|   TEXAS INSTRUMENTS INCORPORATED
|   Standard Linear and Logic
|   IBIS Model of SN74LVTH162241
|   3.3-V ABT 16-BIT BUFFERS/DRIVERS
|   WITH 3-STATE OUTPUTS
|   TSSOP 48-pin package (DGG)
|   SSOP 48-pin package (DL)
[IBIS Ver]   3.2
[Comment char] |_char
[File Name]   sn74lvth162241.ibs
[File Rev]   1.1 | a_die
[Date]   04/12/02
[Source]   File originated at Texas Instruments, Inc
[Notes]   The following is a sample IBIS file for the SNLVTH162241.
   - All test data contained in this file are derived from
   actual measurement.
   - The measurement used DGG package.
   - We have data across voltage and temperature, but not across
   process.
   - Since this is a BiCMOS process, we have irregular trend for the
   curves at high and low temperatures. This data was taken with
   high temperature for strong case and low for weak case.
   - Due to presence of BUS-HOLD at input, GND-CLAMP curves
   have non-monotonic warnings.
   - File created by Nobuhisa Ohtsubo, TIJ SLL Product Engineering.
   - We ommitted some Pwr_Clamp data as there is no Power
   clamp diode at the input
   - Due to 5V tollerant circuitry, we have non-monotonic warnings
   at the pull-up curves
|*   Property of Texas Instruments Incorporated.  Unauthorized   *
|*   reproduction and/or distribution is strictly prohibited.   *
|*   This product is protected under copyright law.   *
|*   Created 1998, (C) Copyright 1998, Texas Instruments Inc.,   *
|*   All Rights Reserved   *
|*   UNLESS THERE IS A SIGNED, WRITTEN AGREEMENT TO THE   *
|*   CONTRARY, TEXAS INSTRUMENTS ("TI") IS PROVIDING THE SPICE   *
|*   MODELS "AS IS" AND WITHOUT ANY WARRANTY, EXPRESSED OR   *
|*   IMPLIED.  TI assumes no liability for:   *
|*   1) the accuracy of the IBIS models provided to your   *
|*   company;   *
|*   2) the proper functioning of these IBIS models in your   *
|*   design or for any resulting applications; or   *
|*   3) infringement of patents, copyrights or intellectual   *
|*   property rights resulting from your use of these   *
|*   IBIS models.   *
|*   TI provides IBIS Models as a service to our customers.   *
|*   You and your company shall not distribute, sell or give   *
|*   these models to anyone else without prior written   *
|*   permission from TI.   *
|*   TI reserves the right to make changes to our products or   *
|*   to discontinue any semiconductor product or service   *
|*   without notice, and advises our customers to obtain the   *
|*   latest version of relevant information to verify, before   *
|*   placing orders, that the information being relied on is   *
|*   current.   *
|*   Please be aware that your receipt and use of the IBIS   *
|*   information provided shall serve as acceptance of these   *
|*   terms and conditions.  If you do not accept these terms,   *
|*   you should return or destroy the IBIS models and any   *
|*   other accompanying information immediately.   *
|   TSSOP PACKAGE (DGG)
[Component]   LVTH162241_DGG
[manufacturer]   Texas Instruments, Inc.
[Package]
|   typ   min   max
R_pkg   0.044   0.038   0.051
L_pkg   3.019nH   2.486nH   4.099nH
C_pkg   0.507pF   0.334pF   0.809pF
[Pin] signal_name   model_name   R_pin   L_pin   C_pin
1   1NOE   LVTH162241_OE   0.041   4.017nH   0.759pF
2   1Y1   LVTH162241_OUT  0.042   3.737nH   0.792pF
3   1Y2   LVTH162241_OUT  0.042   3.48nH   0.661pF
4   GND   GND   0.038   3.131nH   0.575pF
5   1Y3   LVTH162241_OUT  0.047   3.122nH   0.566pF
6   1Y4   LVTH162241_OUT  0.043   2.948nH   0.504pF
7   VCC   POWER   0.045   2.845nH   0.397pF
8   2Y1   LVTH162241_OUT  0.049   2.835nH   0.394pF
9   2Y2   LVTH162241_OUT  0.048   2.715nH   0.378pF
10   GND   GND   0.050   2.664nH   0.363pF
11   2Y3   LVTH162241_OUT  0.050   2.585nH   0.348pF
12   2Y4   LVTH162241_OUT  0.049   2.55nH   0.337pF
13   3Y1   LVTH162241_OUT  0.049   2.541nH   0.336pF
14   3Y2   LVTH162241_OUT  0.050   2.574nH   0.348pF
15   GND   GND   0.049   2.618nH   0.359pF
16   3Y3   LVTH162241_OUT  0.046   2.671nH   0.375pF
17   3Y4   LVTH162241_OUT  0.045   2.754nH   0.389pF
18   VCC   POWER   0.044   2.823nH   0.450pF
19   4Y1   LVTH162241_OUT  0.042   2.968nH   0.503pF
20   4Y2   LVTH162241_OUT  0.051   3.108nH   0.535pF
21   GND   GND   0.042   3.175nH   0.587pF
22   4Y3   LVTH162241_OUT  0.041   3.449nH   0.678pF
23   4Y4   LVTH162241_OUT  0.044   3.766nH   0.804pF
24   4NOE   LVTH162241_OE   0.043   4.065nH   0.761pF
25   3OE   LVTH162241_OE   0.041   3.994nH   0.757pF
26   4A4   LVTH162241_IN   0.039   3.649nH   0.789pF
27   4A3   LVTH162241_IN   0.038   3.362nH   0.660pF
28   GND   GND   0.038   3.082nH   0.574pF
29   4A2   LVTH162241_IN   0.044   2.99nH   0.522pF
30   4A1   LVTH162241_IN   0.041   2.917nH   0.495pF
31   VCC   POWER   0.043   2.82nH   0.448pF
32   3A4   LVTH162241_IN   0.043   2.699nH   0.385pF
33   3A3   LVTH162241_IN   0.045   2.628nH   0.372pF
34   GND   GND   0.046   2.556nH   0.356pF
35   3A2   LVTH162241_IN   0.046   2.495nH   0.344pF
36   3A1   LVTH162241_IN   0.047   2.487nH   0.334pF
37   2A4   LVTH162241_IN   0.047   2.49nH   0.335pF
38   2A3   LVTH162241_IN   0.046   2.486nH   0.343pF
39   GND   GND   0.045   2.566nH   0.356pF
40   2A2   LVTH162241_IN   0.044   2.639nH   0.374pF
41   2A1   LVTH162241_IN   0.043   2.701nH   0.386pF
42   VCC   POWER   0.043   2.817nH   0.450pF
43   1A4   LVTH162241_IN   0.041   2.935nH   0.501pF
44   1A3   LVTH162241_IN   0.047   3.035nH   0.529pF
45   GND   GND   0.043   3.171nH   0.589pF
46   1A2   LVTH162241_IN   0.040   3.415nH   0.682pF
47   1A1   LVTH162241_IN   0.043   3.741nH   0.809pF
48   2OE   LVTH162241_OE   0.044   4.099nH   0.764pF
|   SSOP PACKAGE (DL)
[Component]   LVTH162241_DL
[manufacturer]   Texas Instruments, Inc.
[Package]
|   typ   min   max
R_pkg   0.048   0.038   0.053
L_pkg   6.046nH   5.084nH   7.968nH
C_pkg   0.813pF   0.569pF   1.157pF
[Pin] signal_name   model_name   R_pin   L_pin   C_pin
1   1NOE   LVTH162241_OE   0.046   7.968nH   1.017pF
2   1Y1   LVTH162241_OUT  0.044   7.299nH   1.157pF
3   1Y2   LVTH162241_OUT  0.043   6.765nH   1.058pF
4   GND   GND   0.041   6.269nH   0.933pF
5   1Y3   LVTH162241_OUT  0.038   5.856nH   0.829pF
6   1Y4   LVTH162241_OUT  0.046   5.802nH   0.790pF
7   VCC   POWER   0.050   5.656nH   0.738pF
8   2Y1   LVTH162241_OUT  0.053   5.5nH   0.643pF
9   2Y2   LVTH162241_OUT  0.052   5.304nH   0.606pF
10   GND   GND   0.053   5.189nH   0.583pF
11   2Y3   LVTH162241_OUT  0.051   5.084nH   0.569pF
12   2Y4   LVTH162241_OUT  0.053   5.862nH   0.833pF
13   3Y1   LVTH162241_OUT  0.053   5.862nH   0.833pF
14   3Y2   LVTH162241_OUT  0.051   5.084nH   0.569pF
15   GND   GND   0.053   5.189nH   0.583pF
16   3Y3   LVTH162241_OUT  0.052   5.304nH   0.606pF
17   3Y4   LVTH162241_OUT  0.053   5.5nH   0.643pF
18   VCC   POWER   0.050   5.656nH   0.738pF
19   4Y1   LVTH162241_OUT  0.046   5.802nH   0.790pF
20   4Y2   LVTH162241_OUT  0.038   5.856nH   0.829pF
21   GND   GND   0.041   6.269nH   0.933pF
22   4Y3   LVTH162241_OUT  0.043   6.765nH   1.058pF
23   4Y4   LVTH162241_OUT  0.044   7.299nH   1.157pF
24   4NOE   LVTH162241_OE   0.046   7.968nH   1.017pF
25   3OE   LVTH162241_OE   0.046   7.968nH   1.017pF
26   4A4   LVTH162241_IN   0.044   7.299nH   1.157pF
27   4A3   LVTH162241_IN   0.043   6.765nH   1.058pF
28   GND   GND   0.041   6.269nH   0.933pF
29   4A2   LVTH162241_IN   0.038   5.856nH   0.829pF
30   4A1   LVTH162241_IN   0.046   5.802nH   0.790pF
31   VCC   POWER   0.050   5.656nH   0.738pF
32   3A4   LVTH162241_IN   0.053   5.5nH   0.643pF
33   3A3   LVTH162241_IN   0.052   5.304nH   0.606pF
34   GND   GND   0.053   5.189nH   0.583pF
35   3A2   LVTH162241_IN   0.051   5.084nH   0.569pF
36   3A1   LVTH162241_IN   0.053   5.862nH   0.833pF
37   2A4   LVTH162241_IN   0.053   5.862nH   0.833pF
38   2A3   LVTH162241_IN   0.051   5.084nH   0.569pF
39   GND   GND   0.053   5.189nH   0.583pF
40   2A2   LVTH162241_IN   0.052   5.304nH   0.606pF
41   2A1   LVTH162241_IN   0.053   5.5nH   0.643pF
42   VCC   POWER   0.005   5.656nH   0.738pF
43   1A4   LVTH162241_IN   0.046   5.802nH   0.790pF
44   1A3   LVTH162241_IN   0.038   5.856nH   0.829pF
45   GND   GND   0.041   6.269nH   0.933pF
46   1A2   LVTH162241_IN   0.043   6.765nH   1.058pF
47   1A1   LVTH162241_IN   0.044   7.299nH   1.157pF
48   2OE   LVTH162241_OE   0.046   7.967nH   1.017pF
[Model Selector]   LVTH162241_IN
LVTH162241_IN_28   2.8-V Vcc Input Model
LVTH162241_IN_33   3.3-V Vcc Input Model
[Model Selector]   LVTH162241_OE
LVTH162241_OE_28   2.8-V Vcc Input Model
LVTH162241_OE_33   3.3-V Vcc Input Model
[Model Selector]   LVTH162241_OUT
LVTH162241_OUT_28  2.8-V Vcc Output Model
LVTH162241_OUT_33  3.3-V Vcc Output Model
| Models and submodels in the file (6): LVTH162241_OUT_28 (3-state), LVTH162241_OE_28 (Input), LVTH162241_IN_28 (Input), LVTH162241_OUT_33 (3-state), LVTH162241_OE_33 (Input), LVTH162241_IN_33 (Input)
